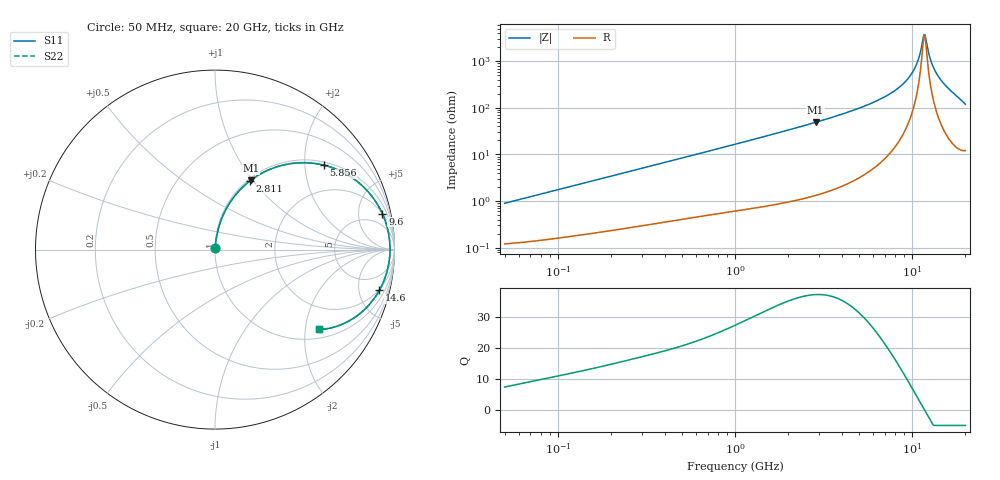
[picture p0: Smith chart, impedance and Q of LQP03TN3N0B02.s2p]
!Murata Part Number: LQP03TN3N0B02
!These Parameters are Measured in Series Mode Connection
!  o--[Z]--o
!Port1  Port2
!  o-------o
!Freq. Start=50[MHz] Stop=20[GHz], 401[Steps]
# Hz S RI R 50
!Freq.(Hz) S11(Real) S11(Imag) S21(Real) S21(Imag) S12(Real) S12(Imag) S22(Real) S22(Imag)
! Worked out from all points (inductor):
!   401 points, 50 MHz to 20 GHz, reference 50 ohm
!   read as one part in series: L = 2.82 nH near 51.52 MHz
!   highest Q = 37.2 at 2.853 GHz (marker M1), where L = 2.74 nH
!   self-resonance near 11.66 GHz
!   S11 on the Smith chart (normalised r, x): 50 MHz: 1.00, +0.02; 2.811 GHz: 1.03, +0.97; 5.856 GHz: 1.09, +2.49; 9.6 GHz: 2.02, +8.94; 14.6 GHz: 1.87, -7.74; 20 GHz: 1.24, -2.38
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5e7  0.00128 0.00886  0.9987 -0.00886  0.9987 -0.00886  0.00128 0.00886
1.364002e8  0.00243 0.0235  0.9976 -0.0235  0.9976 -0.0235  0.00243 0.0235
3.721004e8  0.00724 0.062  0.9928 -0.062  0.9928 -0.062  0.00724 0.062
1e9  0.0322 0.1592  0.9678 -0.1592  0.9678 -0.1592  0.0322 0.1592
1.766834e9  0.0864 0.2665  0.9136 -0.2665  0.9136 -0.2665  0.0864 0.2665
2.728004e9  0.1855 0.3755  0.8145 -0.3755  0.8145 -0.3755  0.1855 0.3755
2.810964e9  0.1954 0.3833  0.8046 -0.3833  0.8046 -0.3833  0.1954 0.3833
2.853386e9  0.2005 0.3872  0.7995 -0.3872  0.7995 -0.3872  0.2005 0.3872
4.026975e9  0.3549 0.4645  0.6451 -0.4645  0.6451 -0.4645  0.3549 0.4645
5.856089e9  0.6047 0.4709  0.3953 -0.4709  0.3953 -0.4709  0.6047 0.4709
7.442007e9  0.7835 0.3865  0.2165 -0.3865  0.2165 -0.3865  0.7835 0.3865
8.644534e9  0.8805 0.2888  0.1195 -0.2888  0.1195 -0.2888  0.8805 0.2888
9.600142e9  0.9322 0.2009  0.0678 -0.2009  0.0678 -0.2009  0.9322 0.2009
1.066139e10  0.9651 0.1002  0.0349 -0.1002  0.0349 -0.1002  0.9651 0.1002
1.149051e10  0.9747 0.023  0.0253 -0.023  0.0253 -0.023  0.9747 0.023
1.166392e10  0.9752 0.00726  0.0248 -0.00726  0.0248 -0.00726  0.9752 0.00726
1.201863e10  0.9744 -0.0245  0.0256 0.0245  0.0256 0.0245  0.9744 -0.0245
1.257102e10  0.9693 -0.0722  0.0307 0.0722  0.0307 0.0722  0.9693 -0.0722
1.314879e10  0.9592 -0.1198  0.0408 0.1198  0.0408 0.1198  0.9592 -0.1198
1.460232e10  0.9156 -0.2272  0.0844 0.2272  0.0844 0.2272  0.9156 -0.2272
1.670968e10  0.8163 -0.349  0.1837 0.349  0.1837 0.349  0.8163 -0.349
2e10  0.5806 -0.4449  0.4194 0.4449  0.4194 0.4449  0.5806 -0.4449
